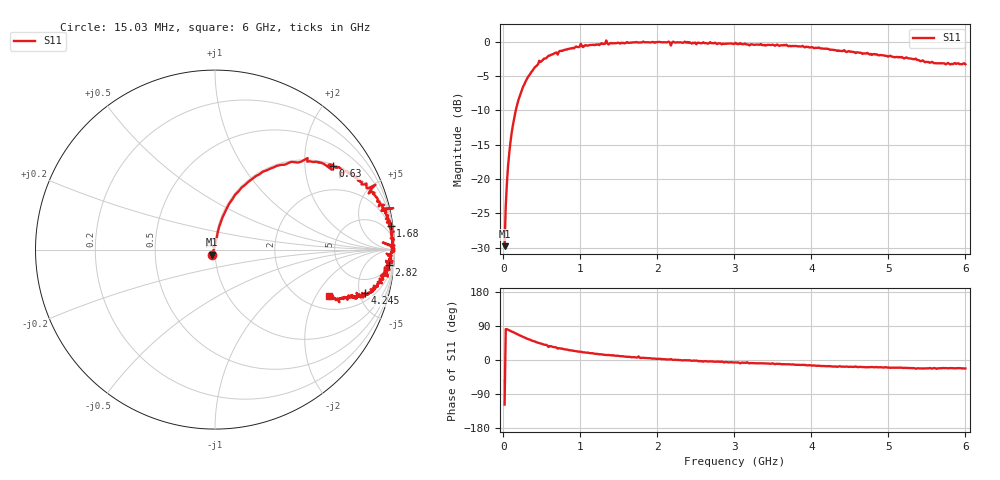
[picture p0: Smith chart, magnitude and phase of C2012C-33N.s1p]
!	Network	Analyzer	HP8753E.07.74:	Oct	30	2002	Serial	No.	JP38451487
!	Hewlett-Packard
!	7	Sep	2009	10:51:08
!	Frequency	S11
#	HZ	S	RI	R	50
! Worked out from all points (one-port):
!   400 points, 15.03 MHz to 6 GHz, reference 50 ohm
!   lowest |S11| = -29.8 dB at 15.03 MHz (marker M1), VSWR 1.07, Z = 48.4 - j2.78 ohm
!   |S11| at or under -10 dB: start of sweep to 160.6 MHz
!   S11 on the Smith chart (normalised r, x): 15.03 MHz: 0.97, -0.06; 630 MHz: 1.05, +2.79; 1.68 GHz: 2, +15; 2.82 GHz: 7, -21; 4.245 GHz: 2.83, -5.63; 6 GHz: 2.64, -2.57
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1.502992e7  -0.015 -0.0287
3.002985e7  0.00929 0.063
6.00297e7  0.0219 0.123
1.050295e8  0.0544 0.206
1.650292e8  0.112 0.305
2.850286e8  0.266 0.434
4.650277e8  0.516 0.51
6.300268e8  0.658 0.465
7.650262e8  0.741 0.427
1.005025e9  0.894 0.361
1.320023e9  0.938 0.229
1.335023e9  0.993 0.231
1.365023e9  0.927 0.217
1.515022e9  0.952 0.171
1.680022e9  0.978 0.13
1.755021e9  0.971 0.162
1.785021e9  0.982 0.0905
2.145019e9  1 0.0217
2.175019e9  0.935 0.0396
2.205019e9  1 0.00403
2.265019e9  0.99 0.00464
2.820016e9  0.967 -0.0839
3.015015e9  0.973 -0.112
3.765011e9  0.909 -0.186
4.245009e9  0.835 -0.243
4.515007e9  0.807 -0.257
5.265004e9  0.705 -0.272
6e9  0.633 -0.259
